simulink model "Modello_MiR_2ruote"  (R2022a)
settings: Solver=VariableStepAuto  StartTime=0.0  StopTime=time_s(end,1)  RelTol=1e-3
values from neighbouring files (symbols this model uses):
  bd = 0.205    [Modello_MiR_2ruote_script.m]    (also in Modello_MiR_6ruote_script.m; Modello_MiR_6ruote_validato_script.m; Modello_MiR_UR_script.m)
  Fx = @(u) (u <= -s2) * (-FL) + (u > -s2 && u <= -s1) * (u*(FL - FLa)/(s2 - s1) + s2*(FL - FLa)/(s2 - s1) - FL) +         + (u > -s1 && u <= s1) * (u * FLa / s1) + (u > s1 && u <= s2) * (u * (FLa - FL)/(s1 - s2) - s2 * (FLa - FL)/(s1 - s2) + FL) +          + (u > s2) * FL    [Modello_MiR_2ruote_script.m]
  Fy = @(u) (u <= -a2) * (-FT) + (u > -a2 && u <= -a1) * (u*(FT - FTa)/(a2 - a1) + a2*(FT - FTa)/(a2 - a1) - FT) +         + (u > -a1 && u <= a1) * (u * FTa / a1) + (u > a1 && u <= a2) * (u * (FTa - FT)/(a1 - a2) - a2 * (FTa - FT)/(a1 - a2) + FT) +          + (u > a2) * FT    [Modello_MiR_2ruote_script.m]
  Idw_1 = 1/2 * mdw * rd^2    (= 0.00551836278784)    [Modello_MiR_2ruote_script.m]    (also in Transfer_Function_Gol_Gcl.m = Inertia_vect(jj,1); Modello_MiR_6ruote_script.m; Modello_MiR_6ruote_validato_script.m; Modello_MiR_UR_script.m)
  iMax = 20.7*1.1    (= 22.77)    [Modello_MiR_2ruote_script.m]    (also in Modello_MiR_6ruote_script.m; Modello_MiR_6ruote_validato_script.m; Modello_MiR_UR_script.m)
  Iv = mv * (l^2 + w^2)  / 12    (= 6.75343333333)    [Modello_MiR_2ruote_script.m]    (also in Modello_MiR_6ruote_script.m; Modello_MiR_6ruote_validato_script.m = 8.95033333333; Modello_MiR_UR_script.m)
  Kc = 0.15    [Modello_MiR_2ruote_script.m]    (also in Modello_MiR_6ruote_script.m; Modello_MiR_6ruote_validato_script.m; Modello_MiR_UR_script.m)
  Ki_i = 1    [Modello_MiR_2ruote_script.m]    (also in Modello_MiR_6ruote_script.m; Modello_MiR_6ruote_validato_script.m; Modello_MiR_UR_script.m)
  Ki_v = 1    [Modello_MiR_2ruote_script.m]    (also in Modello_MiR_6ruote_script.m; Modello_MiR_6ruote_validato_script.m; Modello_MiR_UR_script.m)
  Kp_i = 5    [Modello_MiR_2ruote_script.m]    (also in Modello_MiR_6ruote_script.m; Modello_MiR_6ruote_validato_script.m; Modello_MiR_UR_script.m)
  Kp_v = 5    [Modello_MiR_2ruote_script.m]    (also in Modello_MiR_6ruote_script.m; Modello_MiR_6ruote_validato_script.m; Modello_MiR_UR_script.m)
  L = R * tauE    (= 0.00181134822805)    [Modello_MiR_2ruote_script.m]    (also in Modello_MiR_6ruote_script.m; Modello_MiR_6ruote_validato_script.m; Modello_MiR_UR_script.m)
  mv = 83    [Modello_MiR_2ruote_script.m]    (also in Modello_MiR_6ruote_script.m; Modello_MiR_6ruote_validato_script.m = 110; Modello_MiR_UR_script.m)
  Mz = @(u) (u <= -am2 || u >= am2) * 0 + (u > -am2 && u <= -am1) * (- u * Mza/(am2 -am1) - Mza * am2/(am2 -am1)) +          + (u > -am1 && u <= am1) * (Mza * u / am1) + (u > am1 && u < am2) * (Mza * u /(am1 -am2) - Mza * am2 /(am1 - am2))    [Modello_MiR_2ruote_script.m]
  psi = [psi1;rotation;psi2]    [Modello_MiR_2ruote_script.m]    (also in Modello_MiR_6ruote_script.m; Modello_MiR_6ruote_validato_script.m = psi_interp; Modello_MiR_UR_script.m = psi_interp)
  R = velMax * TorqueMax / (iMax)^2    (= 1.81134822805)    [Modello_MiR_2ruote_script.m]    (also in Modello_MiR_6ruote_script.m; Modello_MiR_6ruote_validato_script.m; Modello_MiR_UR_script.m)
  rap_rid = 10.167    [Modello_MiR_2ruote_script.m]    (also in Modello_MiR_6ruote_script.m; Modello_MiR_6ruote_validato_script.m; Modello_MiR_UR_script.m)
  rd = 0.1    [Modello_MiR_2ruote_script.m]    (also in Modello_MiR_6ruote_script.m; Modello_MiR_6ruote_validato_script.m; Modello_MiR_UR_script.m)
  VaMax = Kc * velMax    (= 41.2443991527)    [Modello_MiR_2ruote_script.m]    (also in Modello_MiR_6ruote_script.m; Modello_MiR_6ruote_validato_script.m; Modello_MiR_UR_script.m)
  X_start = input('Inserire coordinata x iniziale')    [Modello_MiR_2ruote_script.m]    (also in Modello_MiR_6ruote_script.m; Modello_MiR_6ruote_validato_script.m = traj(1,1); Modello_MiR_UR_script.m = traj(1,1))
  Y_start = input('Inserire coordinata y iniziale')    [Modello_MiR_2ruote_script.m]    (also in Modello_MiR_6ruote_script.m; Modello_MiR_6ruote_validato_script.m = traj(1,2); Modello_MiR_UR_script.m = traj(1,2))
libraries: slpidlib x4

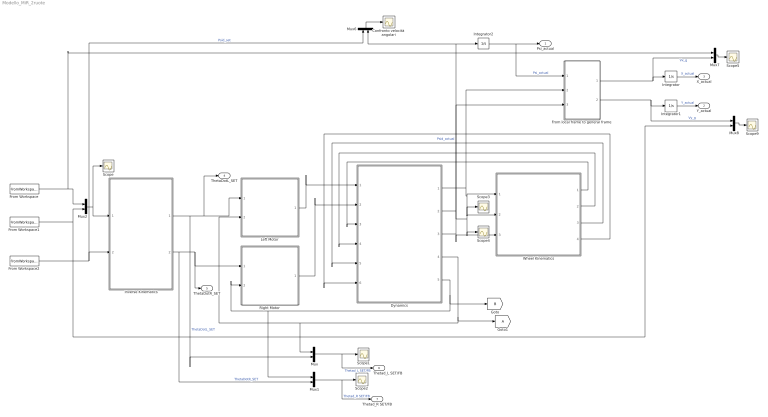
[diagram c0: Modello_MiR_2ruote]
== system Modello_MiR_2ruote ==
  Confronto velocità angolari : Scope
  Dynamics : Subsystem
  From Workspace : FromWorkspace  VariableName=[time_v Xd_set]
  From Workspace1 : FromWorkspace  VariableName=[time_v Yd_set]
  From Workspace2 : FromWorkspace  VariableName=[ time_v psid_set]
  From local frame to general frame : Subsystem
  Goto1 : Goto
  Integrator : Integrator  InitialCondition=X_start
  Integrator1 : Integrator  InitialCondition=Y_start
  Integrator2 : Integrator  InitialCondition=psi(1,1)
  Inverse Kinematics : Subsystem
  Left Motor : Subsystem
  Mux{,1..2,6..8} (6 alike) : Mux  Inputs=2
  Right Motor : Subsystem
  Scope{,1..5,9} (7 alike) : Scope
  Wheel Kinematics : Subsystem
  Psi_actual : Outport
  Y_actual : Outport  Port=2
  X_actual : Outport  Port=3
  ThetaDotL_SET : Outport  Port=4
  ThetaDotR_SET : Outport  Port=5
  Thetad_L SET/FB : Outport  Port=6
  Thetad_R SET/FB : Outport  Port=7
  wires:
  Wheel Kinematics/4(Vy_DR) -> Dynamics/6(Vy_DR)
  Mux7/1 -> Scope5/1
  Mux8/1 -> Scope9/1
  Wheel Kinematics/3(Vx_DR) -> Dynamics/5(Vx_DR)
  Right Motor/1(Cm_R) -> Dynamics/2(Cm_R)
  Dynamics/3(Psid) -> Wheel Kinematics/3(Psid), Mux6/2, Integrator2/1  "Psid_actual"
  Inverse Kinematics/1(ThetaDotL) -> Mux/2, ThetaDotL_SET/1, Left Motor/1(ThetadL_SET)  "ThetaDotL_SET"
  Left Motor/1(Cm_L) -> Dynamics/1(Cm_L)
  Dynamics/2(Vy) -> Wheel Kinematics/2(Vy), Scope4/1, From local frame to general frame/3(Vy)
  Dynamics/5(Thetad_R) -> [B], Mux1/1, Right Motor/2(ThetadR_FB)
  Mux2/1 -> Scope/1, Inverse Kinematics/1(vSet)
  Inverse Kinematics/2(ThetaDotR) -> Mux1/2, ThetaDotR_SET/1, Right Motor/1(ThetadR_SET)  "ThetaDotR_SET"
  From Workspace/1 -> Mux2/1, Mux7/1
  Dynamics/1(Vx) -> Wheel Kinematics/1(Vx), Scope3/1, From local frame to general frame/2(Vx)
  Integrator/1 -> X_actual/1  "X_actual"
  Mux/1 -> Thetad_L SET/FB/1, Scope1/1  "Thetad_L SET/FB"
  From local frame to general frame/1(Vx_g) -> Mux7/2, Integrator/1  "Vx_g"
  Integrator2/1 -> From local frame to general frame/1(Psi), Psi_actual/1  "Psi_actual"
  From local frame to general frame/2(Vy_g) -> Mux8/1, Integrator1/1  "Vy_g"
  Integrator1/1 -> Y_actual/1  "Y_actual"
  Wheel Kinematics/2(Vy_DL) -> Dynamics/4(Vy_DL)
  Mux6/1 -> Confronto velocità angolari/1
  Dynamics/4(Thetad_L) -> Goto1/1, Mux/1, Left Motor/2(ThetadL_FB)
  Wheel Kinematics/1(Vx_DL) -> Dynamics/3(Vx_DL)
  From Workspace1/1 -> Mux2/2, Mux8/2
  From Workspace2/1 -> Inverse Kinematics/2(psiDotSet), Mux6/1  "Psid_set"
  Mux1/1 -> Thetad_R SET/FB/1, Scope2/1  "Thetad_R SET/FB"

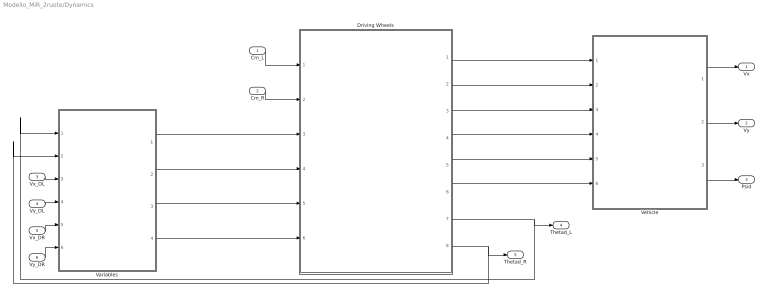
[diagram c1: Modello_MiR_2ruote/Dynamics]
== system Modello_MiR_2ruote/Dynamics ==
  Cm_L : Inport
  Cm_R : Inport  Port=2
  Vx_DL : Inport  Port=3
  Vy_DL : Inport  Port=4
  Vx_DR : Inport  Port=5
  Vy_DR : Inport  Port=6
  Driving Wheels : Subsystem
  Variables : Subsystem
  Vehicle : Subsystem
  Vx : Outport
  Vy : Outport  Port=2
  Psid : Outport  Port=3
  Thetad_L : Outport  Port=4
  Thetad_R : Outport  Port=5
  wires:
  Cm_L/1 -> Driving Wheels/1(Cm_L)
  Cm_R/1 -> Driving Wheels/2(Cm_R)
  Driving Wheels/1(Fx_L) -> Vehicle/1(Fx_L)
  Driving Wheels/2(Fx_R) -> Vehicle/2(Fx_R)
  Driving Wheels/3(Fy_L) -> Vehicle/3(Fy_L)
  Driving Wheels/4(Fy_R) -> Vehicle/4(Fy_R)
  Driving Wheels/5(Mz_L) -> Vehicle/5(Mz_L)
  Driving Wheels/6(Mz_R) -> Vehicle/6(Mz_R)
  Vehicle/2(Vy) -> Vy/1
  Vehicle/1(Vx) -> Vx/1
  Vehicle/3(Psid) -> Psid/1
  Variables/1(Sigma_L) -> Driving Wheels/3(Sigma_L)
  Variables/2(Sigma_R) -> Driving Wheels/4(Sigma_R)
  Variables/3(Alpha_L) -> Driving Wheels/5(Alpha_L)
  Variables/4(Alpha_R) -> Driving Wheels/6(Alpha_R)
  Driving Wheels/7(Thetad_L) -> Thetad_L/1, Variables/1(Thetad_L)
  Driving Wheels/8(Thetad_R) -> Variables/2(Thetad_R), Thetad_R/1
  Vx_DL/1 -> Variables/3(Vx_DL)
  Vy_DL/1 -> Variables/4(Vy_DL)
  Vx_DR/1 -> Variables/5(Vx_DR)
  Vy_DR/1 -> Variables/6(Vy_DR)

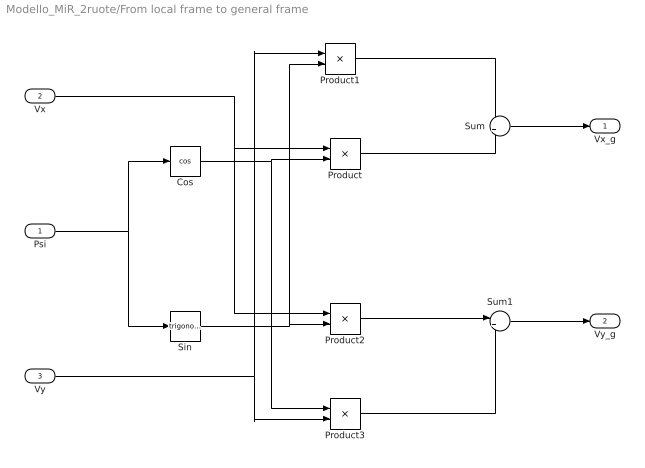
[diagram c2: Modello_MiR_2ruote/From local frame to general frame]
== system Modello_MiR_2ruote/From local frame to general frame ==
  Psi : Inport
  Vx : Inport  Port=2
  Vy : Inport  Port=3
  Cos : Trigonometry  Operator=cos
  Product{,1..3} (4 alike) : Product
  Sin : Trigonometry
  Sum : Sum  Inputs=-+
  Sum1 : Sum  Inputs=|++
  Vx_g : Outport
  Vy_g : Outport  Port=2
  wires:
  Product/1 -> Sum/2
  Sin/1 -> Product2/2, Product1/2
  Product1/1 -> Sum/1
  Vx/1 -> Product2/1, Product/1
  Product2/1 -> Sum1/1
  Cos/1 -> Product3/1, Product/2
  Product3/1 -> Sum1/2
  Psi/1 -> Sin/1, Cos/1
  Vy/1 -> Product3/2, Product1/1
  Sum/1 -> Vx_g/1
  Sum1/1 -> Vy_g/1

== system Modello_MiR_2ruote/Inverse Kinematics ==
  vSet : Inport
  psiDotSet : Inport  Port=2
  Demux : Demux  Outputs=2
  Integrator : Integrator  InitialCondition=pi/2
  MATLAB Function : MATLAB Function  TreatAsAtomicUnit=on
  MATLAB Function1 : MATLAB Function  TreatAsAtomicUnit=on
  Scope1 : Scope
  Scope2 : Scope
  ThetaDotL : Outport
  ThetaDotR : Outport  Port=2
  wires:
  vSet/1 -> Demux/1
  Demux/1 -> MATLAB Function1/2(Xd_set), MATLAB Function/2(Xd_set)  "Xd_set"
  Demux/2 -> MATLAB Function1/3(Yd_set), MATLAB Function/3(Yd_set)  "Yd_set"
  psiDotSet/1 -> MATLAB Function1/4(psid_set), MATLAB Function/4(psid_set), Integrator/1
  Integrator/1 -> MATLAB Function1/1(psi_set), MATLAB Function/1(psi_set)  "Psi_set"
  MATLAB Function/1(Thetad_DR_SET) -> Scope1/1, ThetaDotR/1
  MATLAB Function1/1(Thetad_DL_SET) -> Scope2/1, ThetaDotL/1

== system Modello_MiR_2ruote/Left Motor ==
  ThetadL_SET : Inport
  ThetadL_FB : Inport  Port=2
  Gain : Gain  Gain=rap_rid
  Gain1 : Gain  Gain=rap_rid
  Subsystem : Subsystem
  Subsystem1 : Subsystem
  Cm_L : Outport
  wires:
  Subsystem/1(VaRif) -> Subsystem1/1(VaRif)
  Subsystem1/2(iFB) -> Subsystem/3(iFB)
  ThetadL_SET/1 -> Gain1/1
  ThetadL_FB/1 -> Gain/1
  Subsystem1/1(Torque Cm) -> Cm_L/1
  Gain/1 -> Subsystem1/2(Thetad_FB), Subsystem/2(Thetad_FB)
  Gain1/1 -> Subsystem/1(Thetad_SET)

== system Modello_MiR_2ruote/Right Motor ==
  ThetadR_SET : Inport
  ThetadR_FB : Inport  Port=2
  Gain : Gain  Gain=rap_rid
  Gain1 : Gain  Gain=rap_rid
  Subsystem : Subsystem
  Subsystem1 : Subsystem
  Cm_R : Outport
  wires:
  Subsystem1/2(iFB) -> Subsystem/3(iFB)
  ThetadR_SET/1 -> Gain1/1
  Subsystem/1(VaRif) -> Subsystem1/1(VaRif)
  ThetadR_FB/1 -> Gain/1
  Subsystem1/1(Torque Cm) -> Cm_R/1
  Gain/1 -> Subsystem1/2(Thetad_FB), Subsystem/2(Thetad_FB)
  Gain1/1 -> Subsystem/1(Thetad_SET)

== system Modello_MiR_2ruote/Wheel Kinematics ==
  Vx : Inport
  Vy : Inport  Port=2
  Psid : Inport  Port=3
  Left Wheel : Subsystem
  Right Wheel : Subsystem
  Vx_DL : Outport
  Vy_DL : Outport  Port=2
  Vx_DR : Outport  Port=3
  Vy_DR : Outport  Port=4
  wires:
  Vx/1 -> Right Wheel/1(Vx), Left Wheel/1(Vx)
  Vy/1 -> Right Wheel/2(Vy), Left Wheel/2(Vy)
  Psid/1 -> Right Wheel/3(Psid), Left Wheel/3(Psid)
  Left Wheel/1(Vx_DL) -> Vx_DL/1
  Left Wheel/2(Vy_DL) -> Vy_DL/1
  Right Wheel/1(Vx_DR) -> Vx_DR/1
  Right Wheel/2(Vy_DR) -> Vy_DR/1

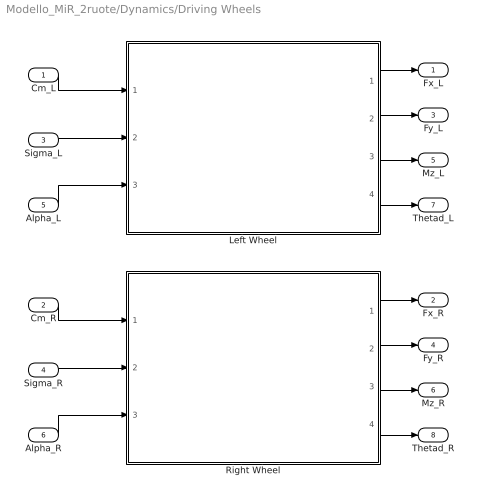
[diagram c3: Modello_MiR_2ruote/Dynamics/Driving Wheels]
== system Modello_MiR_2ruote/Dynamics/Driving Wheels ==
  Cm_L : Inport
  Cm_R : Inport  Port=2
  Sigma_L : Inport  Port=3
  Sigma_R : Inport  Port=4
  Alpha_L : Inport  Port=5
  Alpha_R : Inport  Port=6
  Left Wheel : Subsystem
  Right Wheel : Subsystem
  Fx_L : Outport
  Fx_R : Outport  Port=2
  Fy_L : Outport  Port=3
  Fy_R : Outport  Port=4
  Mz_L : Outport  Port=5
  Mz_R : Outport  Port=6
  Thetad_L : Outport  Port=7
  Thetad_R : Outport  Port=8
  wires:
  Cm_L/1 -> Left Wheel/1(Cm_L)
  Cm_R/1 -> Right Wheel/1(Cm_R)
  Left Wheel/1(Fx_L) -> Fx_L/1
  Right Wheel/1(Fx_R) -> Fx_R/1
  Left Wheel/2(Fy_L) -> Fy_L/1
  Right Wheel/2(Fy_R) -> Fy_R/1
  Right Wheel/3(Mz_R) -> Mz_R/1
  Left Wheel/3(Mz_L) -> Mz_L/1
  Left Wheel/4(Thetad_L) -> Thetad_L/1
  Right Wheel/4(Thetad_R) -> Thetad_R/1
  Sigma_L/1 -> Left Wheel/2(Sigma_L)
  Sigma_R/1 -> Right Wheel/2(Sigma_R)
  Alpha_L/1 -> Left Wheel/3(Alpha_L)
  Alpha_R/1 -> Right Wheel/3(Alpha_R)

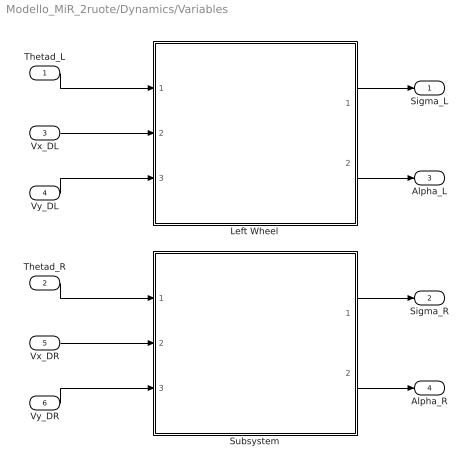
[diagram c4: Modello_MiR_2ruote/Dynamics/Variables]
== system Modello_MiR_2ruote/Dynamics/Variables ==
  Thetad_L : Inport
  Thetad_R : Inport  Port=2
  Vx_DL : Inport  Port=3
  Vy_DL : Inport  Port=4
  Vx_DR : Inport  Port=5
  Vy_DR : Inport  Port=6
  Left Wheel : Subsystem
  Subsystem : Subsystem
  Sigma_L : Outport
  Sigma_R : Outport  Port=2
  Alpha_L : Outport  Port=3
  Alpha_R : Outport  Port=4
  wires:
  Thetad_L/1 -> Left Wheel/1(Thetad_L)
  Vx_DL/1 -> Left Wheel/2(Vx_DL)
  Vy_DL/1 -> Left Wheel/3(Vy_DL)
  Thetad_R/1 -> Subsystem/1(Thetad_R)
  Vx_DR/1 -> Subsystem/2(Vx_DR)
  Vy_DR/1 -> Subsystem/3(Vy_DR)
  Left Wheel/1(Sigma_L) -> Sigma_L/1
  Subsystem/1(Sigma_R) -> Sigma_R/1
  Left Wheel/2(Alpha_L) -> Alpha_L/1
  Subsystem/2(Alpha_R) -> Alpha_R/1

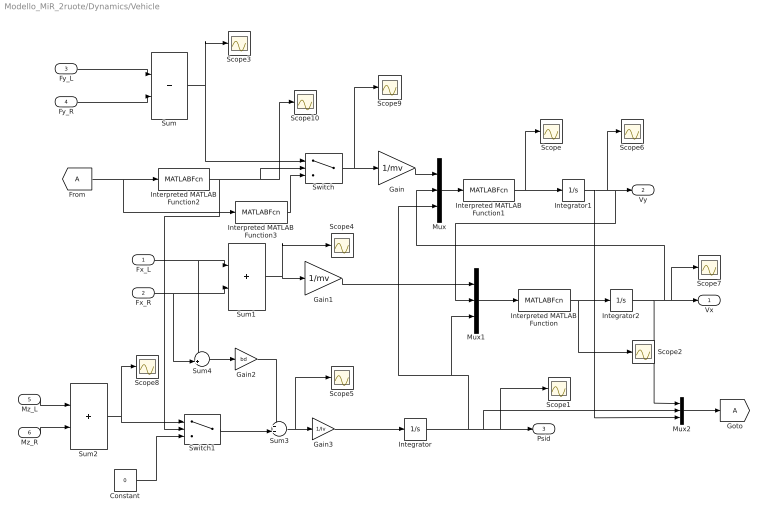
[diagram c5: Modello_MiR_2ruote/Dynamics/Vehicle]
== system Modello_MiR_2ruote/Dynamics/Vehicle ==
  Fx_L : Inport
  Fx_R : Inport  Port=2
  Fy_L : Inport  Port=3
  Fy_R : Inport  Port=4
  Mz_L : Inport  Port=5
  Mz_R : Inport  Port=6
  Constant : Constant  Value=0
  From : From
  Gain : Gain  Gain=1/mv
  Gain1 : Gain  Gain=1/mv
  Gain2 : Gain  Gain=bd
  Gain3 : Gain  Gain=1/Iv
  Goto : Goto
  Integrator : Integrator
  Integrator1 : Integrator
  Integrator2 : Integrator
  Interpreted MATLAB Function : MATLABFcn  MATLABFcn=u(1) + u(2)*u(3)
  Interpreted MATLAB Function1 : MATLABFcn  MATLABFcn=u(1) - u(2)*u(3)
  Interpreted MATLAB Function2 : MATLABFcn  MATLABFcn=(abs(mv*u(1)*u(2))>2*FTa)*1 + (u(3)>0)*1
  Interpreted MATLAB Function3 : MATLABFcn  MATLABFcn=(mv*u(1)*u(2))
  Mux : Mux  Inputs=3
  Mux1 : Mux  Inputs=3
  Mux2 : Mux  Inputs=3
  Scope{,1..10} (11 alike) : Scope
  Sum : Sum
  Sum1 : Sum
  Sum2 : Sum
  Sum3 : Sum  Inputs=++|
  Sum4 : Sum  Inputs=-+|
  Switch : Switch  Criteria=u2 > Threshold
  Switch1 : Switch  Criteria=u2 > Threshold
  Vx : Outport
  Vy : Outport  Port=2
  Psid : Outport  Port=3
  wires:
  Fy_L/1 -> Sum/1
  Fy_R/1 -> Sum/2
  Sum/1 -> Switch/1, Scope3/1
  Sum1/1 -> Scope4/1, Gain1/1
  Fx_R/1 -> Sum4/2, Sum1/2
  Fx_L/1 -> Sum1/1, Sum4/1
  Mz_L/1 -> Sum2/1
  Mz_R/1 -> Sum2/2
  Sum4/1 -> Gain2/1
  Gain2/1 -> Sum3/1
  Sum3/1 -> Scope5/1, Gain3/1
  Gain3/1 -> Integrator/1
  Gain1/1 -> Mux1/1
  Mux/1 -> Interpreted MATLAB Function1/1
  Mux1/1 -> Interpreted MATLAB Function/1
  Integrator2/1 -> Mux2/1, Mux/2, Scope7/1, Vx/1
  Interpreted MATLAB Function/1 -> Integrator2/1, Scope2/1
  Gain/1 -> Mux/1
  Integrator1/1 -> Mux2/3, Mux1/2, Vy/1, Scope6/1
  Interpreted MATLAB Function1/1 -> Integrator1/1, Scope/1
  Switch1/1 -> Sum3/2
  Mux2/1 -> Goto/1
  Integrator/1 -> Mux1/3, Mux/3, Mux2/2, Scope1/1, Psid/1
  Constant/1 -> Switch1/3
  Sum2/1 -> Switch1/1, Scope8/1
  From/1 -> Interpreted MATLAB Function3/1, Interpreted MATLAB Function2/1
  Interpreted MATLAB Function2/1 -> Switch/2, Scope10/1, Switch1/2
  Switch/1 -> Scope9/1, Gain/1
  Interpreted MATLAB Function3/1 -> Switch/3

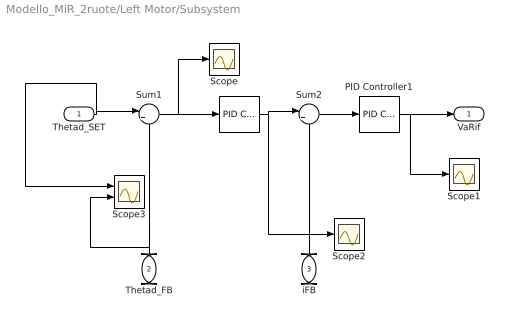
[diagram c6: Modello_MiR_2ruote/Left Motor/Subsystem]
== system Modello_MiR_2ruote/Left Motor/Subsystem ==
  Thetad_SET : Inport
  Thetad_FB : Inport  Port=2
  iFB : Inport  Port=3
  " " : slpidlib/PID Controller  Controller=PID  Form=Parallel  TimeDomain=Continuous-time  UseExternalTs=off  SampleTime=-1  IntegratorMethod=Forward Euler  FilterMethod=Forward Euler  ControllerParametersSource=internal  P=Kp_v  I=Ki_v  UseKiTs=off  D=0  N=1  UseFilter=on  TunerSelectOption=Transfer Function Based (PID Tuner App)  InitialConditionSource=internal  InitialConditionForIntegrator=0  InitialConditionForFilter=0  DifferentiatorICPrevScaledInput=0  ExternalReset=none  TrackingMode=off  Kt=1  LimitOutput=on  SatLimitsSource=internal  UpperSaturationLimit=iMax  LowerSaturationLimit=-iMax  LinearizeAsGain=on  AntiWindupMode=back-calculation  Kb=1  POutMin=[]  POutMax=[]  IOutMin=[]  IOutMax=[]  DOutMin=[]  DOutMax=[]  NOutMin=[]  NOutMax=[]  SumOutMin=[]  SumOutMax=[]  SaturationOutMin=[]  SaturationOutMax=[]  PParamMin=0  PParamMax=[]  IParamMin=0  IParamMax=[]  DParamMin=0  DParamMax=[]  NParamMin=[]  NParamMax=[]  KbParamMin=[]  KbParamMax=[]  KtParamMin=[]  KtParamMax=[]  KbOutMin=[]  KbOutMax=[]  KtOutMin=[]  KtOutMax=[]  IntegratorOutMin=[]  IntegratorOutMax=[]  FilterOutMin=[]  FilterOutMax=[]  SumI1OutMin=[]  SumI1OutMax=[]  SumI2OutMin=[]  SumI2OutMax=[]  SumI3OutMin=[]  SumI3OutMax=[]  SumI4OutMin=[]  SumI4OutMax=[]  SumDOutMin=[]  SumDOutMax=[]  DifferentiatorOutMin=[]  DifferentiatorOutMax=[]  FilterDiffOutCoefMin=[]  FilterDiffOutCoefMax=[]  ReciprocalOutMin=[]  ReciprocalOutMax=[]  SumDenOutMin=[]  SumDenOutMax=[]  SumNumOutMin=[]  SumNumOutMax=[]  DivideOutMin=[]  DivideOutMax=[]  UdiffTsProdOutMin=[]  UdiffTsProdOutMax=[]  NTsProdOutMin=[]  NTsProdOutMax=[]  UintegralTsProdOutMin=[]  UintegralTsProdOutMax=[]  UngainTsProdOutMin=[]  UngainTsProdOutMax=[]  IntegratorContinuousStateAttributes=''  IntegratorStateMustResolveToSignalObject=off  IntegratorRTWStateStorageClass=Auto  FilterContinuousStateAttributes=''  FilterStateMustResolveToSignalObject=off  FilterRTWStateStorageClass=Auto  ParallelPVariant=InternalParameters  IdealPVariant=Disabled  IVariant=InternalParameters  DVariant=InternalParameters  IntegratorVariant=Continuous  SatVariant=Enabled  AWVariant=BackCalculation  PCopyVariant=Disabled  TRVariant=Disabled  FdbkBlocksVariant=Forward  IdealPFdbkVariant=Disabled  SatFdbkVariant=Disabled  DerivativeFilterVariant=ContFilter  NVariant=InternalParameters  NCopyVariant=Disabled  FilterICVariant=InternalICsFilter  IntegratorICVariant=InternalICs  ExternalResetVariant=Disabled  TRSumVariant=Passthrough  SumFdbkVariant=Disabled  SumVariant=Sum_PID  TsampFilterVariant=InternalTs  TsampNgainVariant=Passthrough  TsampIntegralVariant=Passthrough  ExternalSaturationOutDataTypeStr=Inherit: Same as second input  aMode=0
  PID Controller1 : slpidlib/PID Controller  Controller=PID  Form=Parallel  TimeDomain=Continuous-time  UseExternalTs=off  SampleTime=-1  IntegratorMethod=Forward Euler  FilterMethod=Forward Euler  ControllerParametersSource=internal  P=Kp_i  I=Ki_i  UseKiTs=off  D=0  N=100  UseFilter=on  TunerSelectOption=Transfer Function Based (PID Tuner App)  InitialConditionSource=internal  InitialConditionForIntegrator=0  InitialConditionForFilter=0  DifferentiatorICPrevScaledInput=0  ExternalReset=none  TrackingMode=off  Kt=1  LimitOutput=on  SatLimitsSource=internal  UpperSaturationLimit=VaMax  LowerSaturationLimit=-VaMax  LinearizeAsGain=on  AntiWindupMode=back-calculation  Kb=1  POutMin=[]  POutMax=[]  IOutMin=[]  IOutMax=[]  DOutMin=[]  DOutMax=[]  NOutMin=[]  NOutMax=[]  SumOutMin=[]  SumOutMax=[]  SaturationOutMin=[]  SaturationOutMax=[]  PParamMin=[]  PParamMax=[]  IParamMin=[]  IParamMax=[]  DParamMin=[]  DParamMax=[]  NParamMin=[]  NParamMax=[]  KbParamMin=[]  KbParamMax=[]  KtParamMin=[]  KtParamMax=[]  KbOutMin=[]  KbOutMax=[]  KtOutMin=[]  KtOutMax=[]  IntegratorOutMin=[]  IntegratorOutMax=[]  FilterOutMin=[]  FilterOutMax=[]  SumI1OutMin=[]  SumI1OutMax=[]  SumI2OutMin=[]  SumI2OutMax=[]  SumI3OutMin=[]  SumI3OutMax=[]  SumI4OutMin=[]  SumI4OutMax=[]  SumDOutMin=[]  SumDOutMax=[]  DifferentiatorOutMin=[]  DifferentiatorOutMax=[]  FilterDiffOutCoefMin=[]  FilterDiffOutCoefMax=[]  ReciprocalOutMin=[]  ReciprocalOutMax=[]  SumDenOutMin=[]  SumDenOutMax=[]  SumNumOutMin=[]  SumNumOutMax=[]  DivideOutMin=[]  DivideOutMax=[]  UdiffTsProdOutMin=[]  UdiffTsProdOutMax=[]  NTsProdOutMin=[]  NTsProdOutMax=[]  UintegralTsProdOutMin=[]  UintegralTsProdOutMax=[]  UngainTsProdOutMin=[]  UngainTsProdOutMax=[]  IntegratorContinuousStateAttributes=''  IntegratorStateMustResolveToSignalObject=off  IntegratorRTWStateStorageClass=Auto  FilterContinuousStateAttributes=''  FilterStateMustResolveToSignalObject=off  FilterRTWStateStorageClass=Auto  ParallelPVariant=InternalParameters  IdealPVariant=Disabled  IVariant=InternalParameters  DVariant=InternalParameters  IntegratorVariant=Continuous  SatVariant=Enabled  AWVariant=BackCalculation  PCopyVariant=Disabled  TRVariant=Disabled  FdbkBlocksVariant=Forward  IdealPFdbkVariant=Disabled  SatFdbkVariant=Disabled  DerivativeFilterVariant=ContFilter  NVariant=InternalParameters  NCopyVariant=Disabled  FilterICVariant=InternalICsFilter  IntegratorICVariant=InternalICs  ExternalResetVariant=Disabled  TRSumVariant=Passthrough  SumFdbkVariant=Disabled  SumVariant=Sum_PID  TsampFilterVariant=InternalTs  TsampNgainVariant=Passthrough  TsampIntegralVariant=Passthrough  ExternalSaturationOutDataTypeStr=Inherit: Same as second input  aMode=0
  Scope : Scope
  Scope1 : Scope
  Scope2 : Scope
  Scope3 : Scope  NumInputPorts=2
  Sum1 : Sum  Inputs=|+-
  Sum2 : Sum  Inputs=|+-
  VaRif : Outport  VectorParamsAs1DForOutWhenUnconnected=off
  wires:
  Thetad_FB/1 -> Scope3/2, Sum1/2
  " "/1 -> Scope2/1, Sum2/1
  PID Controller1/1 -> Scope1/1, VaRif/1
  iFB/1 -> Sum2/2
  Thetad_SET/1 -> Scope3/1, Sum1/1
  Sum1/1 -> Scope/1, " "/1
  Sum2/1 -> PID Controller1/1

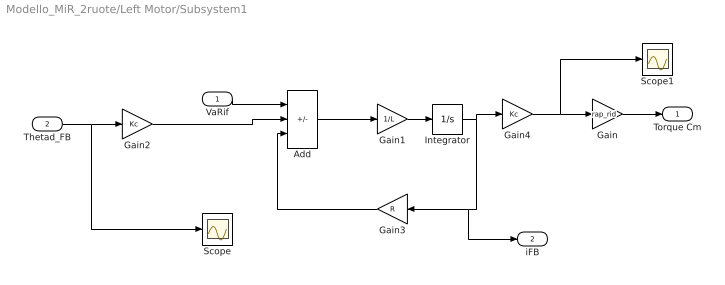
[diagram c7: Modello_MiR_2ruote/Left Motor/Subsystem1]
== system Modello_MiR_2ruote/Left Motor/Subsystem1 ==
  VaRif : Inport
  Thetad_FB : Inport  Port=2
  Add : Sum  Inputs=+--
  Gain : Gain  Gain=rap_rid
  Gain1 : Gain  Gain=1/L
  Gain2 : Gain  Gain=Kc
  Gain3 : Gain  Gain=R
  Gain4 : Gain  Gain=Kc
  Integrator : Integrator
  Scope : Scope
  Scope1 : Scope
  Torque Cm : Outport  VectorParamsAs1DForOutWhenUnconnected=off
  iFB : Outport  Port=2  VectorParamsAs1DForOutWhenUnconnected=off
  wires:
  VaRif/1 -> Add/1
  Add/1 -> Gain1/1
  Gain1/1 -> Integrator/1
  Integrator/1 -> Gain4/1, iFB/1, Gain3/1
  Gain3/1 -> Add/3
  Gain4/1 -> Scope1/1, Gain/1
  Thetad_FB/1 -> Gain2/1, Scope/1
  Gain2/1 -> Add/2
  Gain/1 -> Torque Cm/1

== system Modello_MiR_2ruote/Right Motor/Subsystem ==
  Thetad_SET : Inport
  Thetad_FB : Inport  Port=2
  iFB : Inport  Port=3
  " " : slpidlib/PID Controller  Controller=PID  Form=Parallel  TimeDomain=Continuous-time  UseExternalTs=off  SampleTime=-1  IntegratorMethod=Forward Euler  FilterMethod=Forward Euler  ControllerParametersSource=internal  P=Kp_v  I=Ki_v  UseKiTs=off  D=0  N=1  UseFilter=on  TunerSelectOption=Transfer Function Based (PID Tuner App)  InitialConditionSource=internal  InitialConditionForIntegrator=0  InitialConditionForFilter=0  DifferentiatorICPrevScaledInput=0  ExternalReset=none  TrackingMode=off  Kt=1  LimitOutput=on  SatLimitsSource=internal  UpperSaturationLimit=iMax  LowerSaturationLimit=-iMax  LinearizeAsGain=on  AntiWindupMode=back-calculation  Kb=1  POutMin=[]  POutMax=[]  IOutMin=[]  IOutMax=[]  DOutMin=[]  DOutMax=[]  NOutMin=[]  NOutMax=[]  SumOutMin=[]  SumOutMax=[]  SaturationOutMin=[]  SaturationOutMax=[]  PParamMin=0  PParamMax=[]  IParamMin=0  IParamMax=[]  DParamMin=0  DParamMax=[]  NParamMin=[]  NParamMax=[]  KbParamMin=[]  KbParamMax=[]  KtParamMin=[]  KtParamMax=[]  KbOutMin=[]  KbOutMax=[]  KtOutMin=[]  KtOutMax=[]  IntegratorOutMin=[]  IntegratorOutMax=[]  FilterOutMin=[]  FilterOutMax=[]  SumI1OutMin=[]  SumI1OutMax=[]  SumI2OutMin=[]  SumI2OutMax=[]  SumI3OutMin=[]  SumI3OutMax=[]  SumI4OutMin=[]  SumI4OutMax=[]  SumDOutMin=[]  SumDOutMax=[]  DifferentiatorOutMin=[]  DifferentiatorOutMax=[]  FilterDiffOutCoefMin=[]  FilterDiffOutCoefMax=[]  ReciprocalOutMin=[]  ReciprocalOutMax=[]  SumDenOutMin=[]  SumDenOutMax=[]  SumNumOutMin=[]  SumNumOutMax=[]  DivideOutMin=[]  DivideOutMax=[]  UdiffTsProdOutMin=[]  UdiffTsProdOutMax=[]  NTsProdOutMin=[]  NTsProdOutMax=[]  UintegralTsProdOutMin=[]  UintegralTsProdOutMax=[]  UngainTsProdOutMin=[]  UngainTsProdOutMax=[]  IntegratorContinuousStateAttributes=''  IntegratorStateMustResolveToSignalObject=off  IntegratorRTWStateStorageClass=Auto  FilterContinuousStateAttributes=''  FilterStateMustResolveToSignalObject=off  FilterRTWStateStorageClass=Auto  ParallelPVariant=InternalParameters  IdealPVariant=Disabled  IVariant=InternalParameters  DVariant=InternalParameters  IntegratorVariant=Continuous  SatVariant=Enabled  AWVariant=BackCalculation  PCopyVariant=Disabled  TRVariant=Disabled  FdbkBlocksVariant=Forward  IdealPFdbkVariant=Disabled  SatFdbkVariant=Disabled  DerivativeFilterVariant=ContFilter  NVariant=InternalParameters  NCopyVariant=Disabled  FilterICVariant=InternalICsFilter  IntegratorICVariant=InternalICs  ExternalResetVariant=Disabled  TRSumVariant=Passthrough  SumFdbkVariant=Disabled  SumVariant=Sum_PID  TsampFilterVariant=InternalTs  TsampNgainVariant=Passthrough  TsampIntegralVariant=Passthrough  ExternalSaturationOutDataTypeStr=Inherit: Same as second input  aMode=0
  PID Controller1 : slpidlib/PID Controller  Controller=PID  Form=Parallel  TimeDomain=Continuous-time  UseExternalTs=off  SampleTime=-1  IntegratorMethod=Forward Euler  FilterMethod=Forward Euler  ControllerParametersSource=internal  P=Kp_i  I=Ki_i  UseKiTs=off  D=0  N=100  UseFilter=on  TunerSelectOption=Transfer Function Based (PID Tuner App)  InitialConditionSource=internal  InitialConditionForIntegrator=0  InitialConditionForFilter=0  DifferentiatorICPrevScaledInput=0  ExternalReset=none  TrackingMode=off  Kt=1  LimitOutput=on  SatLimitsSource=internal  UpperSaturationLimit=VaMax  LowerSaturationLimit=-VaMax  LinearizeAsGain=on  AntiWindupMode=back-calculation  Kb=1  POutMin=[]  POutMax=[]  IOutMin=[]  IOutMax=[]  DOutMin=[]  DOutMax=[]  NOutMin=[]  NOutMax=[]  SumOutMin=[]  SumOutMax=[]  SaturationOutMin=[]  SaturationOutMax=[]  PParamMin=[]  PParamMax=[]  IParamMin=[]  IParamMax=[]  DParamMin=[]  DParamMax=[]  NParamMin=[]  NParamMax=[]  KbParamMin=[]  KbParamMax=[]  KtParamMin=[]  KtParamMax=[]  KbOutMin=[]  KbOutMax=[]  KtOutMin=[]  KtOutMax=[]  IntegratorOutMin=[]  IntegratorOutMax=[]  FilterOutMin=[]  FilterOutMax=[]  SumI1OutMin=[]  SumI1OutMax=[]  SumI2OutMin=[]  SumI2OutMax=[]  SumI3OutMin=[]  SumI3OutMax=[]  SumI4OutMin=[]  SumI4OutMax=[]  SumDOutMin=[]  SumDOutMax=[]  DifferentiatorOutMin=[]  DifferentiatorOutMax=[]  FilterDiffOutCoefMin=[]  FilterDiffOutCoefMax=[]  ReciprocalOutMin=[]  ReciprocalOutMax=[]  SumDenOutMin=[]  SumDenOutMax=[]  SumNumOutMin=[]  SumNumOutMax=[]  DivideOutMin=[]  DivideOutMax=[]  UdiffTsProdOutMin=[]  UdiffTsProdOutMax=[]  NTsProdOutMin=[]  NTsProdOutMax=[]  UintegralTsProdOutMin=[]  UintegralTsProdOutMax=[]  UngainTsProdOutMin=[]  UngainTsProdOutMax=[]  IntegratorContinuousStateAttributes=''  IntegratorStateMustResolveToSignalObject=off  IntegratorRTWStateStorageClass=Auto  FilterContinuousStateAttributes=''  FilterStateMustResolveToSignalObject=off  FilterRTWStateStorageClass=Auto  ParallelPVariant=InternalParameters  IdealPVariant=Disabled  IVariant=InternalParameters  DVariant=InternalParameters  IntegratorVariant=Continuous  SatVariant=Enabled  AWVariant=BackCalculation  PCopyVariant=Disabled  TRVariant=Disabled  FdbkBlocksVariant=Forward  IdealPFdbkVariant=Disabled  SatFdbkVariant=Disabled  DerivativeFilterVariant=ContFilter  NVariant=InternalParameters  NCopyVariant=Disabled  FilterICVariant=InternalICsFilter  IntegratorICVariant=InternalICs  ExternalResetVariant=Disabled  TRSumVariant=Passthrough  SumFdbkVariant=Disabled  SumVariant=Sum_PID  TsampFilterVariant=InternalTs  TsampNgainVariant=Passthrough  TsampIntegralVariant=Passthrough  ExternalSaturationOutDataTypeStr=Inherit: Same as second input  aMode=0
  Scope : Scope  NumInputPorts=2
  Sum1 : Sum  Inputs=|+-
  Sum2 : Sum  Inputs=|+-
  VaRif : Outport  VectorParamsAs1DForOutWhenUnconnected=off
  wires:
  Thetad_FB/1 -> Scope/2, Sum1/2
  " "/1 -> Sum2/1
  PID Controller1/1 -> VaRif/1
  iFB/1 -> Sum2/2
  Thetad_SET/1 -> Scope/1, Sum1/1
  Sum1/1 -> " "/1
  Sum2/1 -> PID Controller1/1

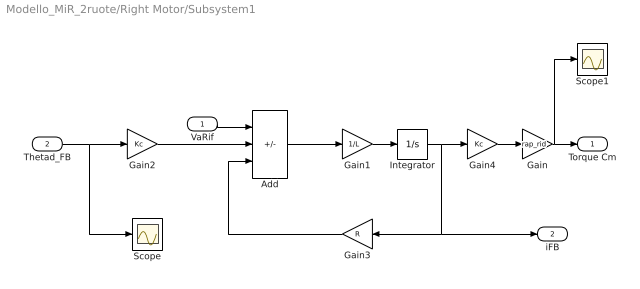
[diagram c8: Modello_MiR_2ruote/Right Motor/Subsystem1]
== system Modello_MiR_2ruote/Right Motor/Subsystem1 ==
  VaRif : Inport
  Thetad_FB : Inport  Port=2
  Add : Sum  Inputs=+--
  Gain : Gain  Gain=rap_rid
  Gain1 : Gain  Gain=1/L
  Gain2 : Gain  Gain=Kc
  Gain3 : Gain  Gain=R
  Gain4 : Gain  Gain=Kc
  Integrator : Integrator
  Scope : Scope
  Scope1 : Scope
  Torque Cm : Outport  VectorParamsAs1DForOutWhenUnconnected=off
  iFB : Outport  Port=2  VectorParamsAs1DForOutWhenUnconnected=off
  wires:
  VaRif/1 -> Add/1
  Add/1 -> Gain1/1
  Gain1/1 -> Integrator/1
  Integrator/1 -> Gain4/1, Gain3/1, iFB/1
  Gain3/1 -> Add/3
  Thetad_FB/1 -> Gain2/1, Scope/1
  Gain2/1 -> Add/2
  Gain4/1 -> Gain/1
  Gain/1 -> Scope1/1, Torque Cm/1

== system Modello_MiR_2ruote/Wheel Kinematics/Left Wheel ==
  Vx : Inport
  Vy : Inport  Port=2
  Psid : Inport  Port=3
  Interpreted MATLAB Function : MATLABFcn  MATLABFcn=u(1) - u(3)*bd
  Interpreted MATLAB Function1 : MATLABFcn  MATLABFcn=u(2)
  Mux : Mux  Inputs=3
  Scope : Scope
  Vx_DL : Outport
  Vy_DL : Outport  Port=2
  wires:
  Vy/1 -> Mux/2
  Vx/1 -> Mux/1
  Psid/1 -> Mux/3
  Mux/1 -> Interpreted MATLAB Function1/1, Interpreted MATLAB Function/1
  Interpreted MATLAB Function1/1 -> Vy_DL/1
  Interpreted MATLAB Function/1 -> Scope/1, Vx_DL/1

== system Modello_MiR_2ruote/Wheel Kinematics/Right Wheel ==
  Vx : Inport
  Vy : Inport  Port=2
  Psid : Inport  Port=3
  Interpreted MATLAB Function : MATLABFcn  MATLABFcn=u(1) + u(3)*bd
  Interpreted MATLAB Function1 : MATLABFcn  MATLABFcn=u(2)
  Mux : Mux  Inputs=3
  Scope : Scope
  Vx_DR : Outport
  Vy_DR : Outport  Port=2
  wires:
  Vy/1 -> Mux/2
  Vx/1 -> Mux/1
  Psid/1 -> Mux/3
  Mux/1 -> Interpreted MATLAB Function/1, Interpreted MATLAB Function1/1
  Interpreted MATLAB Function/1 -> Scope/1, Vx_DR/1
  Interpreted MATLAB Function1/1 -> Vy_DR/1

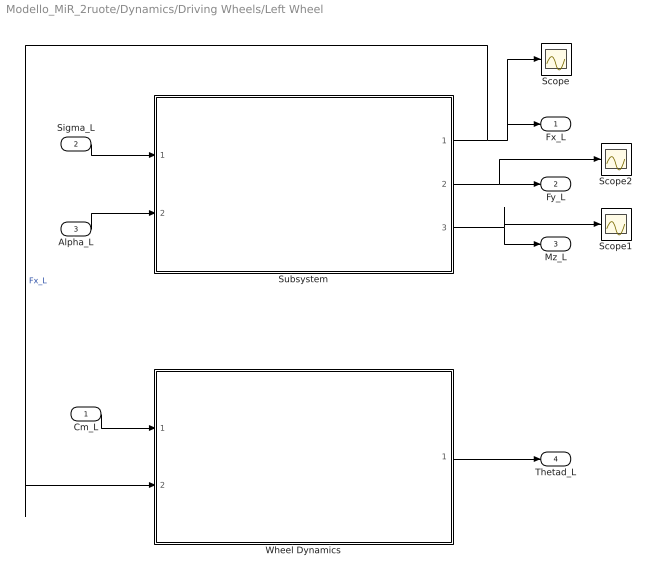
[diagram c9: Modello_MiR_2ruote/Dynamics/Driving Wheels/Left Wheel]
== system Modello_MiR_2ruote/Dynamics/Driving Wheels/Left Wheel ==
  Cm_L : Inport
  Sigma_L : Inport  Port=2
  Alpha_L : Inport  Port=3
  Scope : Scope
  Scope1 : Scope
  Scope2 : Scope
  Subsystem : Subsystem
  Wheel Dynamics : Subsystem
  Fx_L : Outport
  Fy_L : Outport  Port=2
  Mz_L : Outport  Port=3
  Thetad_L : Outport  Port=4
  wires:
  Cm_L/1 -> Wheel Dynamics/1(Cm_L)
  Wheel Dynamics/1(Thetad_L) -> Thetad_L/1
  Sigma_L/1 -> Subsystem/1(Sigma_L)
  Alpha_L/1 -> Subsystem/2(Alpha_L)
  Subsystem/1(Fx_L) -> Scope/1, Fx_L/1, Wheel Dynamics/2(Fx_L)  "Fx_L"
  Subsystem/2(Fy_L) -> Scope2/1, Fy_L/1
  Subsystem/3(Mz_L) -> Scope1/1, Mz_L/1

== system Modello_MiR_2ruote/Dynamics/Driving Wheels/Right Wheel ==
  Cm_R : Inport
  Sigma_R : Inport  Port=2
  Alpha_R : Inport  Port=3
  Scope : Scope
  Scope1 : Scope
  Scope2 : Scope
  Subsystem : Subsystem
  Subsystem1 : Subsystem
  Fx_R : Outport
  Fy_R : Outport  Port=2
  Mz_R : Outport  Port=3
  Thetad_R : Outport  Port=4
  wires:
  Cm_R/1 -> Subsystem/1(Cm_R)
  Alpha_R/1 -> Subsystem1/2(Alpha_R)
  Sigma_R/1 -> Subsystem1/1(Sigma_R)
  Subsystem1/1(Fx_R) -> Scope/1, Fx_R/1, Subsystem/2(Fx_R)
  Subsystem1/2(Fy_R) -> Scope1/1, Fy_R/1
  Subsystem1/3(Mz_R) -> Scope2/1, Mz_R/1
  Subsystem/1(Thetad_R) -> Thetad_R/1

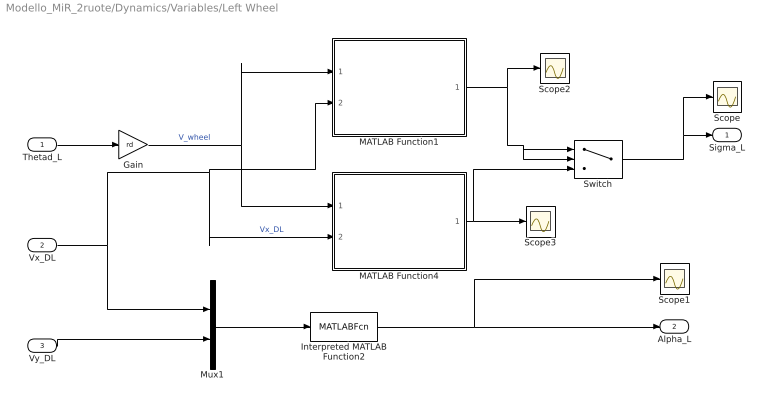
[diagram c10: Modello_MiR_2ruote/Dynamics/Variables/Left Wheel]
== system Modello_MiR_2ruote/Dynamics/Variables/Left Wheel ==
  Thetad_L : Inport
  Vx_DL : Inport  Port=2
  Vy_DL : Inport  Port=3
  Gain : Gain  Gain=rd
  Interpreted MATLAB Function2 : MATLABFcn  MATLABFcn=asin(u(2)/((u(1)^2+u(2)^2)^0.5+1*(((u(1)^2+u(2)^2)^0.5)==0)))
  MATLAB Function1 : MATLAB Function  TreatAsAtomicUnit=on
  MATLAB Function4 : MATLAB Function  TreatAsAtomicUnit=on
  Mux1 : Mux  Inputs=2
  Scope{,1..3} (4 alike) : Scope
  Switch : Switch
  Sigma_L : Outport
  Alpha_L : Outport  Port=2
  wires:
  Thetad_L/1 -> Gain/1
  Vx_DL/1 -> MATLAB Function4/2(Vx_DL), MATLAB Function1/2(Vx_DL), Mux1/1  "Vx_DL"
  Vy_DL/1 -> Mux1/2
  Gain/1 -> MATLAB Function4/1(v_wheel), MATLAB Function1/1(v_wheel)  "V_wheel"
  Mux1/1 -> Interpreted MATLAB Function2/1
  Interpreted MATLAB Function2/1 -> Scope1/1, Alpha_L/1
  Switch/1 -> Scope/1, Sigma_L/1
  MATLAB Function1/1(Fc_pos_out) -> Scope2/1, Switch/1, Switch/2
  MATLAB Function4/1(Fc_neg_out) -> Switch/3, Scope3/1

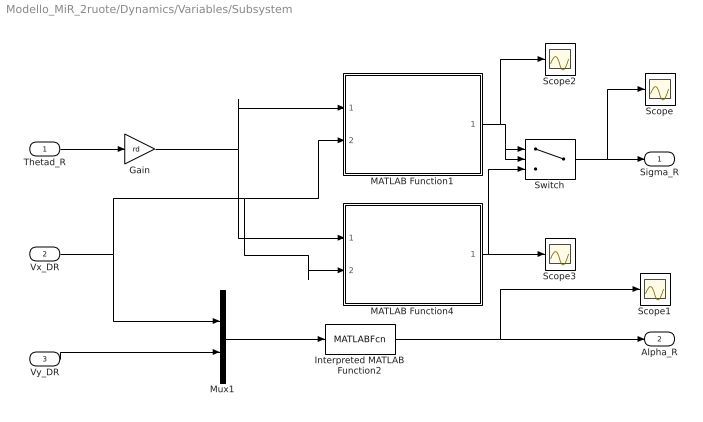
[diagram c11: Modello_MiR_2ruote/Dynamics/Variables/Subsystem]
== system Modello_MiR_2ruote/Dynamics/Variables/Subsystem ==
  Thetad_R : Inport
  Vx_DR : Inport  Port=2
  Vy_DR : Inport  Port=3
  Gain : Gain  Gain=rd
  Interpreted MATLAB Function2 : MATLABFcn  MATLABFcn=asin(u(2)/((u(1)^2+u(2)^2)^0.5+1*(((u(1)^2+u(2)^2)^0.5)==0)))
  MATLAB Function1 : MATLAB Function  TreatAsAtomicUnit=on
  MATLAB Function4 : MATLAB Function  TreatAsAtomicUnit=on
  Mux1 : Mux  Inputs=2
  Scope{,1..3} (4 alike) : Scope
  Switch : Switch
  Sigma_R : Outport
  Alpha_R : Outport  Port=2
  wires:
  Vy_DR/1 -> Mux1/2
  Vx_DR/1 -> MATLAB Function4/2(Vx_DR), MATLAB Function1/2(Vx_DR), Mux1/1
  Interpreted MATLAB Function2/1 -> Scope1/1, Alpha_R/1
  Thetad_R/1 -> Gain/1
  Mux1/1 -> Interpreted MATLAB Function2/1
  Switch/1 -> Scope/1, Sigma_R/1
  Gain/1 -> MATLAB Function4/1(v_wheel), MATLAB Function1/1(v_wheel)
  MATLAB Function1/1(Fc_pos_out) -> Scope2/1, Switch/2, Switch/1
  MATLAB Function4/1(Fc_neg_out) -> Scope3/1, Switch/3

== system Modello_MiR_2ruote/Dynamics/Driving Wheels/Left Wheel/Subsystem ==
  Sigma_L : Inport
  Alpha_L : Inport  Port=2
  Gain : Gain  Gain=-1
  Interpreted MATLAB Function : MATLABFcn  MATLABFcn=Fx(u)
  Interpreted MATLAB Function1 : MATLABFcn  MATLABFcn=Mz(u)
  Interpreted MATLAB Function2 : MATLABFcn  MATLABFcn=Fy(u)
  Fx_L : Outport
  Fy_L : Outport  Port=2
  Mz_L : Outport  Port=3
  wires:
  Sigma_L/1 -> Interpreted MATLAB Function/1
  Interpreted MATLAB Function/1 -> Fx_L/1
  Alpha_L/1 -> Interpreted MATLAB Function1/1, Interpreted MATLAB Function2/1
  Interpreted MATLAB Function2/1 -> Gain/1
  Gain/1 -> Fy_L/1
  Interpreted MATLAB Function1/1 -> Mz_L/1

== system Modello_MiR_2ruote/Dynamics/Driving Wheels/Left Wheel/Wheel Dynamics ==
  Cm_L : Inport
  Fx_L : Inport  Port=2
  Gain : Gain  Gain=rd
  Gain1 : Gain  Gain=1/(Idw_1+2*10^(-3))
  Integrator : Integrator
  Interpreted MATLAB Function : MATLABFcn  MATLABFcn=mv*9.806/6*(kk*u+kv*u^2+cccc*(u==0))
  Scope : Scope
  Sum : Sum  Inputs=+--
  Thetad_L : Outport
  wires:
  Cm_L/1 -> Sum/1
  Gain/1 -> Sum/2
  Interpreted MATLAB Function/1 -> Sum/3
  Integrator/1 -> Interpreted MATLAB Function/1, Thetad_L/1
  Sum/1 -> Scope/1, Gain1/1
  Gain1/1 -> Integrator/1
  Fx_L/1 -> Gain/1

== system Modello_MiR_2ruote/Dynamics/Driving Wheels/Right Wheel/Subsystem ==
  Cm_R : Inport
  Fx_R : Inport  Port=2
  Gain : Gain  Gain=rd
  Gain1 : Gain  Gain=1/(Idw_1+2*10^(-3))
  Integrator : Integrator
  Interpreted MATLAB Function : MATLABFcn  MATLABFcn=mv*9.806/6*(kk*u+kv*u^2+cccc*(u==0))
  Mux : Mux  Inputs=3
  Scope : Scope
  Sum : Sum  Inputs=+--
  Thetad_R : Outport
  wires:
  Interpreted MATLAB Function/1 -> Mux/2, Sum/3  "Res_rot"
  Gain/1 -> Mux/3, Sum/2  "rd*Fc_R"
  Sum/1 -> Gain1/1
  Gain1/1 -> Integrator/1
  Integrator/1 -> Thetad_R/1, Interpreted MATLAB Function/1
  Fx_R/1 -> Gain/1
  Cm_R/1 -> Mux/1, Sum/1  "Cm_R"
  Mux/1 -> Scope/1

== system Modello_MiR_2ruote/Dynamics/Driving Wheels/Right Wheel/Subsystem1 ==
  Sigma_R : Inport
  Alpha_R : Inport  Port=2
  Gain : Gain  Gain=-1
  Interpreted MATLAB Function : MATLABFcn  MATLABFcn=Fx(u)
  Interpreted MATLAB Function1 : MATLABFcn  MATLABFcn=Mz(u)
  Interpreted MATLAB Function2 : MATLABFcn  MATLABFcn=Fy(u)
  Fx_R : Outport
  Fy_R : Outport  Port=2
  Mz_R : Outport  Port=3
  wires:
  Sigma_R/1 -> Interpreted MATLAB Function/1
  Alpha_R/1 -> Interpreted MATLAB Function1/1, Interpreted MATLAB Function2/1
  Gain/1 -> Fy_R/1
  Interpreted MATLAB Function1/1 -> Mz_R/1
  Interpreted MATLAB Function/1 -> Fx_R/1
  Interpreted MATLAB Function2/1 -> Gain/1

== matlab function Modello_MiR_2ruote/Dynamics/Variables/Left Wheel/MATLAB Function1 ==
function Fc_pos_out = fcn(v_wheel,Vx_DL)
x = v_wheel;

y = Vx_DL;

cccc = 1e20;

Fc_pos = @(x,y) ((((x-y)/abs(x+1/cccc))*(((x-y)/abs(x+1/cccc))<=1 )+ 1*(((x-y)/abs(x+1/cccc))>1))*(x*y>=0 && x>=0) + (((x-y)/abs(y+1/cccc))*(((x-y)/abs(y+1/cccc))<=1 ))*(x*y>0 && x<0)+ (x*y<0)*(x/abs(x+1/cccc)))*(0.02<(x^2+y^2)) + (10*(x-y)*(10*(x-y)<1) +1*(10*(x-y)>=1))*(0.02>=(x^2+y^2));

Fc_pos_out = Fc_pos(x,y);

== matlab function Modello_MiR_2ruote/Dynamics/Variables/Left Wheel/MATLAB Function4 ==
function Fc_neg_out = fcn(v_wheel,Vx_DL)
x=v_wheel;

y=Vx_DL;

cccc=1e20;

Fc_neg=@(x,y) ((((x-y)/abs(y+1/cccc))*(((x-y)/abs(y+1/cccc))>=-1)+ (-1)*(((x-y)/abs(y+1/cccc))<-1))*(x*y>=0 && y>=0) + (((x-y)/abs(x+1/cccc))*(((x-y)/abs(x+1/cccc))>=-1))*(x*y>0 && y<0) + (x*y<0)*(x/abs(x+1/cccc)) )*(0.02<(x^2+y^2)) +(10*(x-y)*(10*(x-y)>-1) -1*(10*(x-y)<=-1))*(0.02>=(x^2+y^2)); 

Fc_neg_out = Fc_neg(x,y);

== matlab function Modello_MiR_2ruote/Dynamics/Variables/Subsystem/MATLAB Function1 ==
function Fc_pos_out = fcn(v_wheel,Vx_DR)

x = v_wheel;

y = Vx_DR;

cccc = 1e20;

Fc_pos = @(x,y) ((((x-y)/abs(x+1/cccc))*(((x-y)/abs(x+1/cccc))<=1 )+ 1*(((x-y)/abs(x+1/cccc))>1))*(x*y>=0 && x>=0) + (((x-y)/abs(y+1/cccc))*(((x-y)/abs(y+1/cccc))<=1 ))*(x*y>0 && x<0)+ (x*y<0)*(x/abs(x+1/cccc)))*(0.02<(x^2+y^2)) + (10*(x-y)*(10*(x-y)<1) +1*(10*(x-y)>=1))*(0.02>=(x^2+y^2));


Fc_pos_out = Fc_pos(x,y);

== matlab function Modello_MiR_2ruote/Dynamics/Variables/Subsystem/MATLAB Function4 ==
function Fc_neg_out = fcn(v_wheel,Vx_DR)

x = v_wheel;

y = Vx_DR;

cccc = 1e20;

Fc_neg = @(x,y) ((((x-y)/abs(y+1/cccc))*(((x-y)/abs(y+1/cccc))>=-1)+ (-1)*(((x-y)/abs(y+1/cccc))<-1))*(x*y>=0 && y>=0) + (((x-y)/abs(x+1/cccc))*(((x-y)/abs(x+1/cccc))>=-1))*(x*y>0 && y<0) + (x*y<0)*(x/abs(x+1/cccc)) )*(0.02<(x^2+y^2)) +(10*(x-y)*(10*(x-y)>-1) -1*(10*(x-y)<=-1))*(0.02>=(x^2+y^2)); 


Fc_neg_out = Fc_neg(x,y);

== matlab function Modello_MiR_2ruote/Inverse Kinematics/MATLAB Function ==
function Thetad_DR_SET = angvelR(psi_set, Xd_set, Yd_set, psid_set)
 bd = 0.2050;
 rd = 0.1;
Thetad_DR_SET = 1/rd * (Xd_set * cos(psi_set) + Yd_set * sin(psi_set) + bd*psid_set);

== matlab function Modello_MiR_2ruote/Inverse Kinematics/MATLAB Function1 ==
function Thetad_DL_SET = angvelL(psi_set, Xd_set, Yd_set, psid_set)
 bd = 0.2050;
 rd = 0.1;
Thetad_DL_SET = 1/rd * (Xd_set * cos(psi_set) + Yd_set * sin(psi_set) - bd*psid_set);
